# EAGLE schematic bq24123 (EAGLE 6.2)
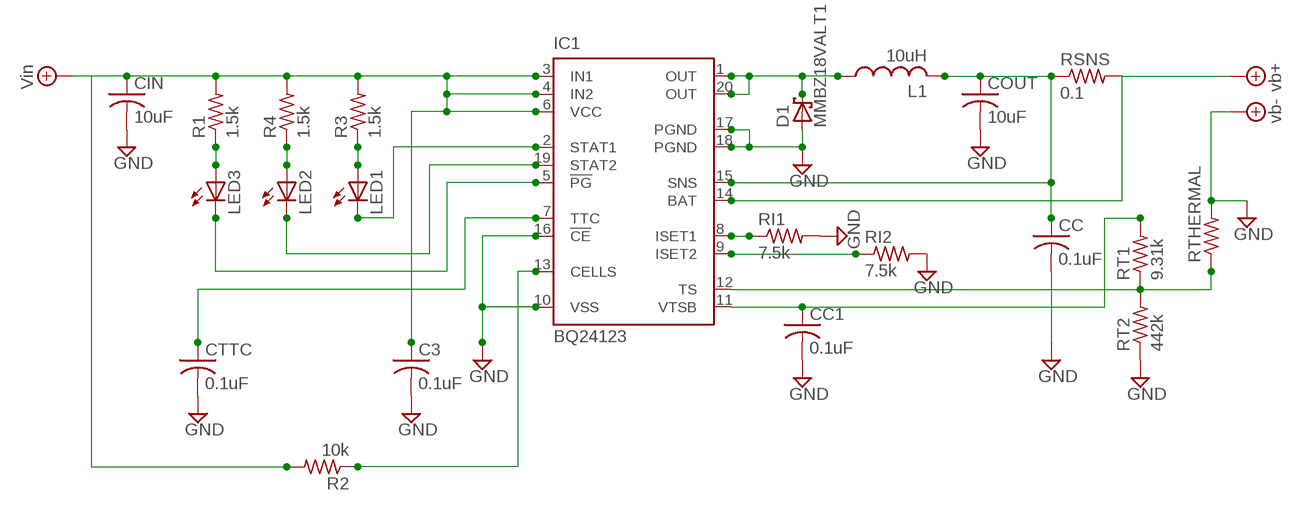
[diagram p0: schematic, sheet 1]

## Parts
C3  0.1uF  C-US025-025X050  [C025-025X050]
CC  0.1uF  C-US025-025X050  [C025-025X050]
CC1  0.1uF  C-US025-025X050  [C025-025X050]
CIN  10uF  C-US025-025X050  [C025-025X050]
COUT  10uF  C-US025-025X050  [C025-025X050]
CTTC  0.1uF  C-US025-025X050  [C025-025X050]
D1  MMBZ18VALT1  1N5908  [C4111-15]
IC1  BQ24123  [QFN20_3,5X4,5]
L1  10uH  L-US0204/5  [0204/5]
LED1  LYW57B  [W57B]
LED2  LYW57B  [W57B]
LED3  LYW57B  [W57B]
R1  1.5k  R-US_0204/2V  [0204V]
R2  10k  R-US_0204/2V  [0204V]
R3  1.5k  R-US_0204/2V  [0204V]
R4  1.5k  R-US_0204/2V  [0204V]
RI1  7.5k  R-US_0204/2V  [0204V]
RI2  7.5k  R-US_0204/2V  [0204V]
RSNS  0.1  R-US_0204/2V  [0204V]
RT1  9.31k  R-US_0204/2V  [0204V]
RT2  442k  R-US_0204/2V  [0204V]
RTHERMAL  R-US_0204/2V  [0204V]

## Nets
+4.1V: C3.1 CIN.1 IC1.3(IN1) IC1.4(IN2) IC1.6(VCC) IC1.14(BAT) R1.2 R2.2 R3.2 R4.2 RSNS.2 RTHERMAL.2 ; supply symbol labelled GND, vb-, vb+, Vin
GND: C3.2 CC1.2 CC.2 CIN.2 COUT.2 CTTC.2 D1.A IC1.10(VSS) IC1.16(!CE) IC1.17(PGND) IC1.18(PGND) RI1.2 RI2.2 RT2.1
N$1: D1.C IC1.1(OUT) IC1.20(OUT) L1.1
N$2: CC.1 COUT.1 IC1.15(SNS) L1.2 RSNS.1
N$4: IC1.8(ISET1) RI1.1
N$5: IC1.9(ISET2) RI2.1
N$6: IC1.12(TS) RT1.1 RT2.2 RTHERMAL.1
N$7: CC1.1 IC1.11(VTSB) RT1.2
N$8: LED3.A R1.1
N$9: LED2.A R4.1
N$10: LED1.A R3.1
N$11: IC1.2(STAT1) LED1.C LED1.C@1(C) LED1.C@2(C) LED1.C@3(C) LED1.C@4(C) LED1.C@5(C)
N$12: IC1.19(STAT2) LED2.C LED2.C@1(C) LED2.C@2(C) LED2.C@3(C) LED2.C@4(C) LED2.C@5(C)
N$13: IC1.5(!PG) LED3.C LED3.C@1(C) LED3.C@2(C) LED3.C@3(C) LED3.C@4(C) LED3.C@5(C)
N$14: CTTC.1 IC1.7(TTC)
N$15: IC1.13(CELLS) R2.1
Unconnected: IC1.EXP IC1.EXP@1 IC1.EXP@2 IC1.EXP@3 IC1.EXP@4 IC1.EXP@5 IC1.EXP@6 IC1.EXP@7 IC1.EXP@8 IC1.EXP@9 IC1.EXP@10 IC1.EXP@11 IC1.EXP@12

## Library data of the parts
C3 CC CC1 CIN COUT CTTC = resistor:C-US: CAPACITOR, American symbol
D1 = diode:1N5908: DIODE
IC1 = texas:BQ24123: SINGLE-CHIP SWITCHMODE, LI-ION AND LI-POLYMER CHARGE-MANAGEMENT IC WITH ENHANCED EMI PERFORMANCE(bqSWITCHER) Source: www.ti.com .. TI-bq24125.pdf; MPN: BQ24123RHLT; OC_FARNELL: 1407131; OC_NEWARK: 84K0851
L1 = resistor:L-US: INDUCTOR, American symbol
LED1-LED3 = led:*W57B: Golden Dragon® 1 Watt LED
R1-R4 RI1 RI2 RSNS RT1 RT2 RTHERMAL = resistor:R-US_: RESISTOR, American symbol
